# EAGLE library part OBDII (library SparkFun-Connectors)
OBD-II Connector OBDII is an on board diagnostics standard that is used on a large variety of cars. Here is the connector we sell at SparkFun: OBD-II connector (DEV-09911) Info and Pinout (sorry, no datasheet) We do not use this connector on any active designs, however, if you're looking for OBDII tech, please check out these: SparkFun OBD related products
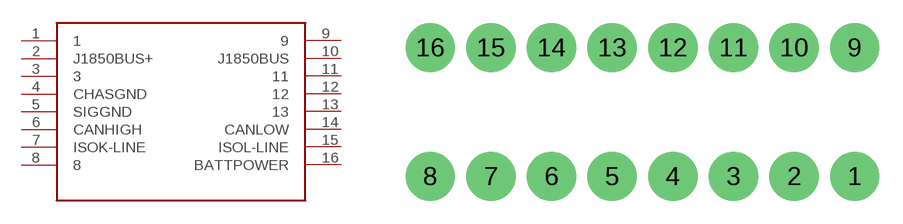
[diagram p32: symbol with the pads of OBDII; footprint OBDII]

Designator prefix J

## OBDII (SF_ID: DEV-09911)  [OBDII]
1  1
2  J1850BUS+
3  3
4  CHASGND
5  SIGGND
6  CANHIGH
7  ISOK-LINE
8  8
9  9
10  J1850BUS
11  11
12  12
13  13
14  CANLOW
15  ISOL-LINE
16  BATTPOWER

## Footprint OBDII (pad centres in mm)
OBD-II Automotive Connector Specifications: Pin count: 16 Pin pitch:0.15" Example device(s): OBD-II
drill 2.2: 1 13.68,-3.81; 2 9.73,-3.81; 3 5.78,-3.81; 4 1.83,-3.81; 5 -2.12,-3.81; 6 -6.07,-3.81; 7 -10.02,-3.81; 8 -13.97,-3.81; 9 13.68,4.59; 10 9.73,4.59; 11 5.78,4.59; 12 1.83,4.59; 13 -2.12,4.59; 14 -6.07,4.59; 15 -10.02,4.59; 16 -13.97,4.59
